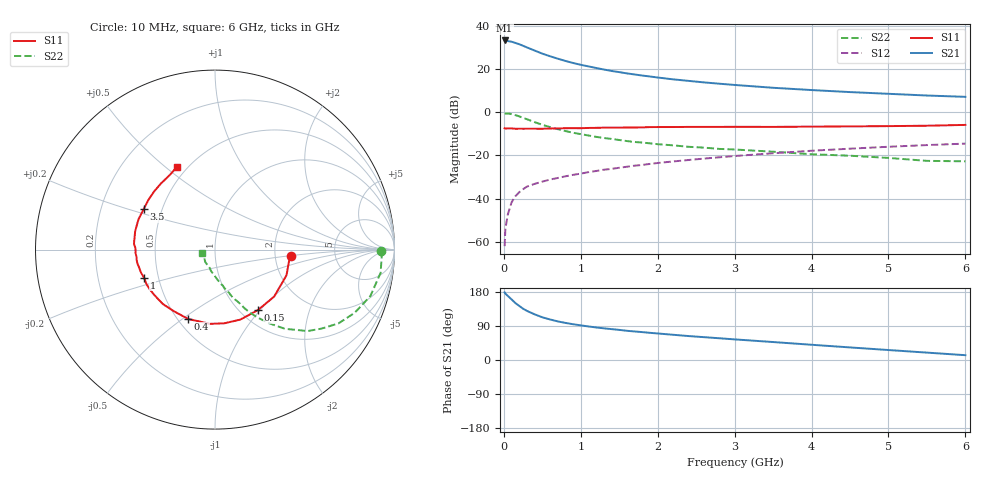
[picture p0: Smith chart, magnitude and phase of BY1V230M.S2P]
! SIEMENS Small Signal Semiconductors
! BFY420
! Si NPN RF SIEGET Grounded Emitter Transistor in MICRO-X
! VCE = 1.25 V  IC = 30 mA
! Common Emitter S-Parameters:  October  1996
# GHz  S  MA  R  50
!  f  S11  S21  S12  S22
! GHz  MAG  ANG  MAG  ANG  MAG  ANG  MAG  ANG
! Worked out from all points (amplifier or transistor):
!   36 points, 10 MHz to 6 GHz, reference 50 ohm
!   highest |S21| = 33.1 dB at 10 MHz (marker M1)
!   |S21| within 3 dB of that: start of sweep to 285.6 MHz
!   unconditionally stable (mu >= 1): start of sweep to 13.67 MHz; 1.461 GHz to end of sweep
!   at 250 MHz: K = 0.39, MSG = 33.1 dB, |S12| = -35.6 dB
!   at 1.4 GHz: K = 0.99, MSG = 22.6 dB, |S12| = -26.2 dB
!   at 6 GHz: K = 1.08, MAG = 9.1 dB, |S12| = -14.5 dB
!   S11 on the Smith chart (normalised r, x): 10 MHz: 2.45, -0.22; 150 MHz: 1.20, -0.97; 400 MHz: 0.56, -0.53; 1 GHz: 0.42, -0.16; 3.5 GHz: 0.39, +0.22; 6 GHz: 0.44, +0.55
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0.01  0.4233 -4.9  45.41 178.5  0.0008 114.6  0.9236 -0.6
0.02  0.4176 -8.2  45.07 175.2  0.002 87.5  0.9295 -2.4
0.05  0.4232 -19.7  44 169.4  0.0042 87.5  0.9318 -8.0
0.1  0.421 -38.4  42.48 160.0  0.0082 75.7  0.9034 -16.7
0.15  0.4131 -54.7  39.8 150.2  0.0114 69.8  0.8539 -24.4
0.2  0.4147 -70.1  37.2 142.8  0.0141 68.7  0.8011 -30.9
0.25  0.4139 -82.7  34.15 135.4  0.0166 63.2  0.7386 -36.6
0.3  0.4146 -93.7  31.37 129.6  0.019 63.9  0.6874 -41.3
0.4  0.4145 -111.1  26.54 120.5  0.022 59.8  0.5882 -48.6
0.5  0.413 -124.3  22.51 112.7  0.0248 58.2  0.5107 -53.6
0.6  0.42 -133.8  19.6 107.0  0.0277 58.2  0.4519 -57.5
0.7  0.4216 -142.3  17.25 101.9  0.0301 57.9  0.4051 -60.8
0.8  0.4256 -148.3  15.27 97.9  0.0329 57.8  0.3659 -63.3
1  0.4253 -158.5  12.43 91.4  0.038 58.4  0.3107 -66.9
1.1  0.4318 -162.7  11.42 88.5  0.0411 59.2  0.2889 -69.3
1.4  0.4402 -172.0  8.962 81.5  0.0489 59.3  0.2407 -73.7
1.6  0.4432 -177.6  7.868 77.1  0.0548 58.8  0.2148 -76.8
2.2  0.4533 170.9  5.736 66.6  0.0726 56.5  0.1711 -84.7
3.5  0.4568 150.5  3.66 47.4  0.1123 48.0  0.122 -100.3
4.5  0.4689 136.3  2.911 33.2  0.1433 38.9  0.0985 -113.4
5.5  0.4859 121.2  2.425 19.5  0.1734 29.0  0.0749 -143.6
6  0.5076 114.6  2.26 12.7  0.1877 23.8  0.0732 -165.5
